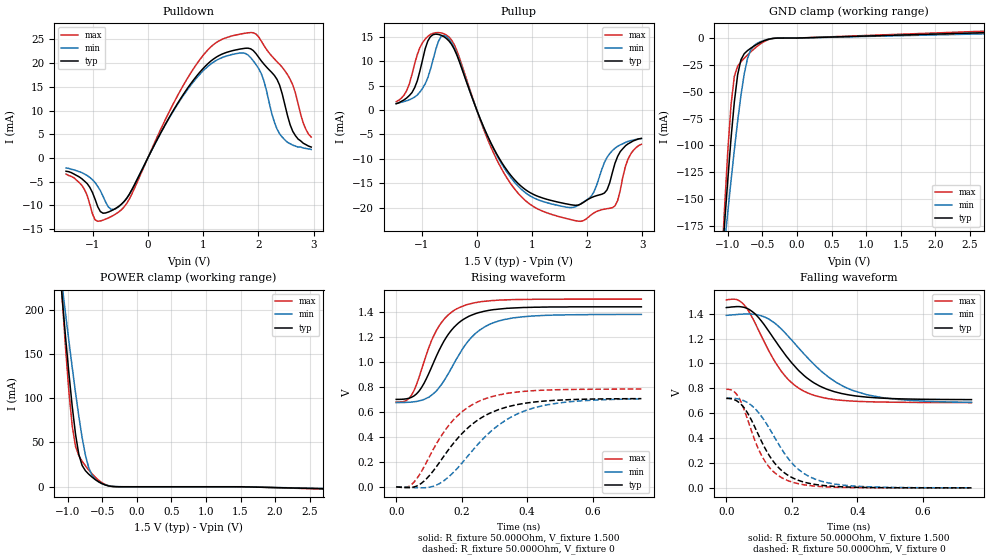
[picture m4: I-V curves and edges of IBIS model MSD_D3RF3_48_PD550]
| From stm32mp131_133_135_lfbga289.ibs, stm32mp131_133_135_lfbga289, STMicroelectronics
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[Model] MSD_D3RF3_48_PD550
Model_type   I/O
C_comp 2.415pF   2.332pF   2.538pF
Vinh = 925.000mV
Vinl = 575.000mV
Vmeas = 750.000mV
Vref = 750.000mV
[Model Spec]
Vinh   925.000mV   888.000mV   963.000mV
Vinl   575.000mV   538.000mV   613.000mV
Vmeas   750.000mV   713.000mV   788.000mV
Vref   750.000mV   713.000mV   788.000mV
[Temperature Range]   25.000   125.000   -40.000
[Voltage Range]   1.500V   1.425V   1.575V
[GND Clamp Reference]   0.00V   0.00V   0.00V
[Pulldown Reference]   0.00V   0.00V   0.00V
[POWER Clamp Reference]   1.500V   1.425V   1.575V
[Pullup Reference]   1.500V   1.425V   1.575V
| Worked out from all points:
|   slope of the pulldown table from 0 to 0.225 V, typ, clamps not added: 44.1 ohm
|   slope of the pullup table from 0 to 0.225 V, typ, clamps not added: 37.5 ohm
|   GND clamp passes 1 mA (typ) near -0.40 V on its own axis
|   POWER clamp passes 1 mA (typ) near -0.41 V on its own axis
|   rising waveform, R_fixture 50.000Ohm, V_fixture 1.500: 20-80 % time 93.7ps typ, 110ps min, 79.6ps max; typ from 0.701 V to 1.45 V
|   rising waveform, R_fixture 50.000Ohm, V_fixture 0: 20-80 % time 151ps typ, 170ps min, 130ps max; typ from -0.003 V to 0.707 V
|   falling waveform, R_fixture 50.000Ohm, V_fixture 1.500: 20-80 % time 142ps typ, 171ps min, 114ps max; typ from 1.45 V to 0.709 V
|   falling waveform, R_fixture 50.000Ohm, V_fixture 0: 20-80 % time 96.6ps typ, 115ps min, 80ps max; typ from 0.719 V to 0 V
[GND Clamp]
-1.48V    -594.8mA   -480.6mA   -764.4mA
-1.098V   -218.9mA   -223.9mA   -221.1mA
-1.05V    -174.6mA   -192.8mA   -160.4mA
-1.002V   -132.4mA   -162.4mA   -105.9mA
-954.6mV  -93.31mA   -132.8mA   -62.14mA
-906.8mV  -59.46mA   -104.2mA   -35.71mA
-859.1mV  -34.19mA   -77.49mA   -26.14mA
-811.4mV  -20.25mA   -53.36mA   -22.06mA
-715.9mV  -11.67mA   -18.95mA   -15.74mA
-572.7mV  -5.563mA   -4.762mA   -7.514mA
-286.4mV  -72.83uA   -122.9uA   -58.2uA
2.959V    5.427mA    4.273mA    6.977mA
[Power Clamp]
-1.459V   578.6mA    479.9mA    724.1mA
-1.077V   211.6mA    226mA      211mA
-1.03V    168.7mA    195.1mA    156.2mA
-981.8mV  128mA      164.7mA    107.3mA
-934.1mV  90.94mA    135mA      68.85mA
-886.4mV  59.42mA    106.5mA    45.71mA
-838.6mV  36.53mA    79.7mA     35.09mA
-743.2mV  18.14mA    35.77mA    23.67mA
-647.7mV  10.94mA    13mA       14.59mA
-552.3mV  5.6mA      5.535mA    7.379mA
-313.6mV  101uA      237.7uA    117.6uA
2.98V     -2.761mA   -2.315mA   -3.352mA
[Pulldown]
-1.48V    -2.8mA     -2.1mA     -3.4mA
-1.193V   -4.4mA     -3.1mA     -5.8mA
-954.6mV  -8.71mA    -5.2mA     -13.05mA
-811.4mV  -11.65mA   -8.07mA    -13.12mA
-525mV    -10.19mA   -10.29mA   -11.37mA
906.8mV   17.62mA    17.19mA    20.18mA
1.766V    23.15mA    22.04mA    26.31mA
2.052V    20.52mA    17.86mA    24.7mA
2.386V    15.37mA    5.1mA      19.75mA
2.625V    5.6mA      2.7mA      15.4mA
2.816V    3.1mA      2.1mA      7.3mA
2.959V    2.3mA      1.8mA      4.4mA
[Pullup]
-1.459V   1.3mA      1.357mA    1.729mA
-1.173V   3.6mA      2.371mA    7.343mA
-981.8mV  10.3mA     4.457mA    13.83mA
-838.6mV  15.06mA    8.354mA    15.51mA
-552.3mV  14.7mA     15.09mA    15.38mA
640.9mV   -13.71mA   -14.18mA   -15.51mA
1.834V    -19.47mA   -19.55mA   -22.76mA
2.12V     -17.72mA   -16.78mA   -21.08mA
2.311V    -16.99mA   -10.74mA   -20.29mA
2.502V    -10.9mA    -7.814mA   -19.63mA
2.741V    -6.9mA     -6.386mA   -9.986mA
2.98V     -5.8mA     -5.843mA   -7.014mA
[Ramp]
R_load=50.000Ohm
dV/dt_r   433.830mV/123.000ps  422.879mV/141.000ps  482.070mV/105.500ps
dV/dt_f   433.830mV/119.000ps  422.879mV/144.000ps  482.070mV/97.500ps
[Rising waveform]
R_fixture=50.000Ohm
V_fixture=1.500
V_fixture_min=1.425
V_fixture_max=1.575
0s        700.9mV    674.8mV    679.3mV
31ps      705.3mV    676.6mV    691.8mV
46ps      716.6mV    679.2mV    731.4mV
77ps      794.2mV    693.4mV    937mV
108ps     959.5mV    734.7mV    1.174V
146ps     1.17V      850.1mV    1.345V
199ps     1.333V     1.091V     1.446V
253ps     1.399V     1.254V     1.484V
330ps     1.431V     1.343V     1.501V
749ps     1.445V     1.384V     1.507V
[Rising waveform]
R_fixture=50.000Ohm
V_fixture=0
0s        -3.056mV   -1.78mV    -3.354mV
31ps      -8.596mV   -5.328mV   -6.146mV
54ps      -4.036mV   -8.681mV   34.02mV
85ps      43.64mV    -10.33mV   158.1mV
131ps     189.6mV    21.92mV    379.6mV
199ps     420.3mV    182.6mV    597.1mV
268ps     565mV      390.6mV    702.1mV
337ps     638.5mV    537.6mV    748mV
429ps     681.6mV    638.5mV    772.1mV
749ps     706.8mV    704.5mV    783.9mV
[Falling waveform]
R_fixture=50.000Ohm
V_fixture=1.500
V_fixture_min=1.425
V_fixture_max=1.575
0s        1.449V     1.387V     1.511V
31ps      1.457V     1.393V     1.514V
54ps      1.451V     1.397V     1.472V
85ps      1.405V     1.395V     1.34V
131ps     1.254V     1.355V     1.095V
184ps     1.056V     1.233V     885.6mV
253ps     870.6mV    1.032V     758.4mV
337ps     768.3mV    845.8mV    707.7mV
429ps     729.2mV    748.7mV    692.6mV
749ps     709.4mV    687.3mV    685.2mV
[Falling waveform]
R_fixture=50.000Ohm
V_fixture=0
0s        719mV      720.5mV    792.7mV
23ps      710.3mV    719.4mV    775.9mV
39ps      685.6mV    713.2mV    721.6mV
85ps      499.7mV    643.5mV    396.8mV
108ps     371mV      572.1mV    258.1mV
131ps     260.3mV    479.5mV    166.2mV
184ps     108.6mV    253.6mV    62.59mV
238ps     45.75mV    114.3mV    24.51mV
322ps     13.16mV    34.83mV    6.049mV
749ps     100.7uV    274uV      -1.98uV
